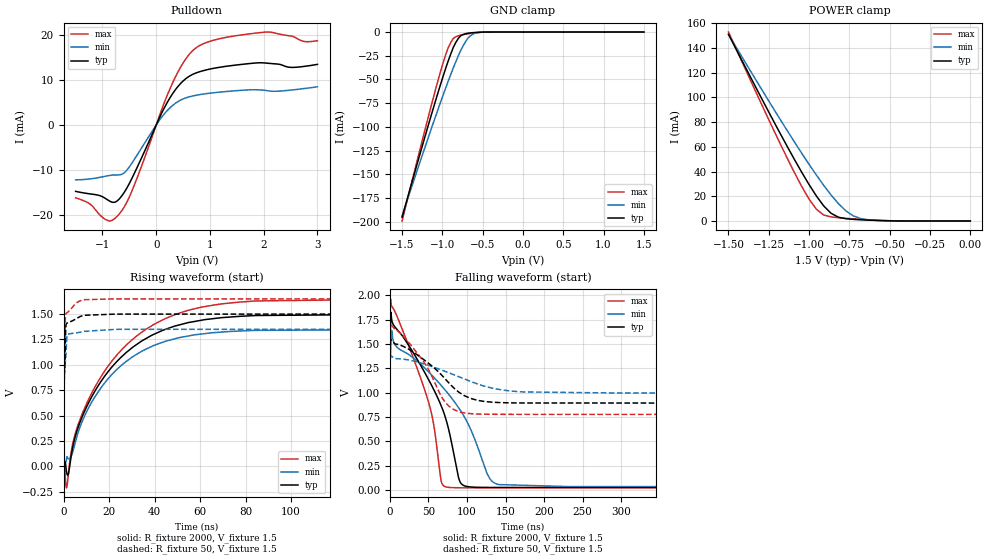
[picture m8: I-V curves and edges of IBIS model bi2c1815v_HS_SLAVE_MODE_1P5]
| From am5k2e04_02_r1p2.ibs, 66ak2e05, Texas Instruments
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|   Model Cell bi2c1815v_HS_SLAVE_MODE_1P5
|bi2c1815gfzhsv.ibs   [11Jan12 revision 1.0]
|bi2c1815v_HS_SLAVE_MODE_1P5
[Model]   bi2c1815v_HS_SLAVE_MODE_1P5
Model_type   I/O_open_drain
Polarity   Non-Inverting
Enable   Active-Low
Vinl =  0.45
Vinh =  1.05
Cref =  15.0000pF
Rref =  100.0000M
Vref =  1.5
Vmeas =  0.75
C_comp   7.63862p   2.44169p   8.22121p
[Model Spec]
Vinl   0.45   0.405   0.495
Vinh   1.05   0.945   1.155
[Temperature Range]   25   125   -40
[Voltage Range]   1.5   1.35   1.65
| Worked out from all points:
|   slope of the pulldown table from 0 to 0.225 V, typ, clamps not added: 41.5 ohm
|   GND clamp passes 1 mA (typ) near -0.66 V on its own axis
|   POWER clamp passes 1 mA (typ) near -0.68 V on its own axis
|   rising waveform, R_fixture 2000, V_fixture 1.5: 20-80 % time 26.9ns typ, 25ns min, 29.1ns max; typ from 0.027 V to 1.5 V
|   rising waveform, R_fixture 50, V_fixture 1.5: 20-80 % time 397ps typ, 478ps min, 363ps max; typ from 0.894 V to 1.5 V
|   falling waveform, R_fixture 2000, V_fixture 1.5: 20-80 % time 38.8ns typ, 55.1ns min, 30.4ns max; typ from 1.5 V to 0.027 V
|   falling waveform, R_fixture 50, V_fixture 1.5: 20-80 % time 50.6ns typ, 71.8ns min, 38.9ns max; typ from 1.5 V to 0.894 V
[POWER_clamp]
|   voltage   I(typ)   I(min)   I(max)
-1.5V     151mA      150.9mA    152.8mA
-1.273V   93.69mA    101.9mA    88.24mA
-1.091V   49.77mA    63.93mA    39.17mA
-1V       29.43mA    45.82mA    17.67mA
-939.4mV  17.53mA    34.37mA    7.927mA
-909.1mV  12.18mA    28.82mA    4.843mA
-863.6mV  6.238mA    21.05mA    3.309mA
-818.2mV  3.071mA    14.07mA    2.668mA
-727.3mV  1.364mA    4.256mA    1.737mA
-681.8mV  1.02mA     2.019mA    1.336mA
-500mV    171uA      194.3uA    230.4uA
0V        214.9pA    5.588nA    92.86pA
[Pulldown]
|   voltage   I(typ)   I(min)   I(max)
-1.5V     -14.74mA   -12.19mA   -16.16mA
-1.227V   -15.31mA   -11.97mA   -17.6mA
-909.1mV  -16.6mA    -11.3mA    -21.18mA
-681.8mV  -16.35mA   -11.08mA   -19.67mA
-454.5mV  -11.91mA   -8.507mA   -14.74mA
272.7mV   6.362mA    3.997mA    8.501mA
545.5mV   10.24mA    5.996mA    14.59mA
772.7mV   11.69mA    6.665mA    17.39mA
1.227V    12.9mA     7.352mA    19.28mA
2.045V    13.75mA    7.657mA    20.64mA
2.5V      12.79mA    7.745mA    19.78mA
3V        13.46mA    8.49mA     18.71mA
[GND_clamp]
|   voltage   I(typ)   I(min)   I(max)
-1.5V     -195.5mA   -194.1mA   -199.3mA
-1.227V   -113.8mA   -124.5mA   -107mA
-1.045V   -61.55mA   -79.59mA   -48.43mA
-954.5mV  -37.21mA   -58.07mA   -22.7mA
-893.9mV  -22.74mA   -44.36mA   -10.65mA
-863.6mV  -16.14mA   -37.7mA    -6.624mA
-803mV    -6.914mA   -25.34mA   -4.002mA
-772.7mV  -3.892mA   -19.56mA   -3.316mA
-712.1mV  -1.754mA   -10.17mA   -2.298mA
-651.5mV  -919.5uA   -3.984mA   -1.444mA
-590.9mV  -443.7uA   -1.105mA   -766.2uA
1.5V      214.9pA    164.2nA    51.75pA
[Ramp]
| variable   typ   min   max
dV/dt_f   0.3897/55.606268n   0.228138/78.172156n   0.561498/43.170448n
dV/dt_r 32.222987m/0.13279357n 18.826586m/0.17051445n 47.234798m/0.1197675n
R_load = 50
[Rising Waveform]
R_fixture = 2000
V_fixture = 1.5
V_fixture_min = 1.35
V_fixture_max = 1.65
|   time   V(typ)   V(min)   V(max)
0s        27.04mV    36.49mV    23.38mV
474.5ps   28.24mV    36.41mV    24.24mV
1.328ns   -55.83mV   81.33mV    -210.5mV
2.182ns   -70.72mV   74.52mV    -61.38mV
4.38ns    226mV      170.3mV    258.5mV
9.583ns   560.6mV    512.9mV    590.6mV
31ns      1.184V     1.089V     1.265V
54.02ns   1.413V     1.282V     1.533V
84.73ns   1.486V     1.34V      1.63V
1.25us    1.5V       1.35V      1.65V
[Rising Waveform]
R_fixture = 50
V_fixture = 1.5
V_fixture_min = 1.35
V_fixture_max = 1.65
|   time   V(typ)   V(min)   V(max)
0s        893.7mV    997mV      778.5mV
383.2ps   912.9mV    999.6mV    841.3mV
452.8ps   925.3mV    1.002V     923.9mV
565ps     969.8mV    1.006V     1.135V
717.3ps   1.125V     1.017V     1.4V
954.7ps   1.354V     1.058V     1.499V
1.396ns   1.41V      1.26V      1.511V
1.609ns   1.412V     1.297V     1.514V
9.023ns   1.488V     1.33V      1.642V
1.25us    1.5V       1.35V      1.65V
[Falling Waveform]
R_fixture = 2000
V_fixture = 1.5
V_fixture_min = 1.35
V_fixture_max = 1.65
|   time   V(typ)   V(min)   V(max)
0s        1.5V       1.35V      1.65V
588ps     1.643V     1.351V     1.949V
1.265ns   1.824V     1.519V     1.917V
37.83ns   1.309V     1.309V     1.195V
54.99ns   1.061V     1.175V     748.8mV
66.7ns    862mV      1.073V     86.62mV
73.38ns   708.1mV    1.011V     31.28mV
92.65ns   64.82mV    803.3mV    23.74mV
140.8ns   27.14mV    57.16mV    23.4mV
1.25us    27.04mV    36.49mV    23.41mV
[Falling Waveform]
R_fixture = 50
V_fixture = 1.5
V_fixture_min = 1.35
V_fixture_max = 1.65
|   time   V(typ)   V(min)   V(max)
0s        1.5V       1.35V      1.65V
962.7ps   1.543V     1.376V     1.713V
37.14ns   1.379V     1.312V     1.388V
49.19ns   1.308V     1.283V     1.251V
65.28ns   1.196V     1.238V     982.1mV
74.9ns    1.113V     1.209V     874.4mV
102ns     949.5mV    1.124V     786.7mV
131.7ns   902.9mV    1.048V     778.4mV
172.6ns   894.4mV    1.008V     777.8mV
1.25us    893.7mV    997mV      777.8mV
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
